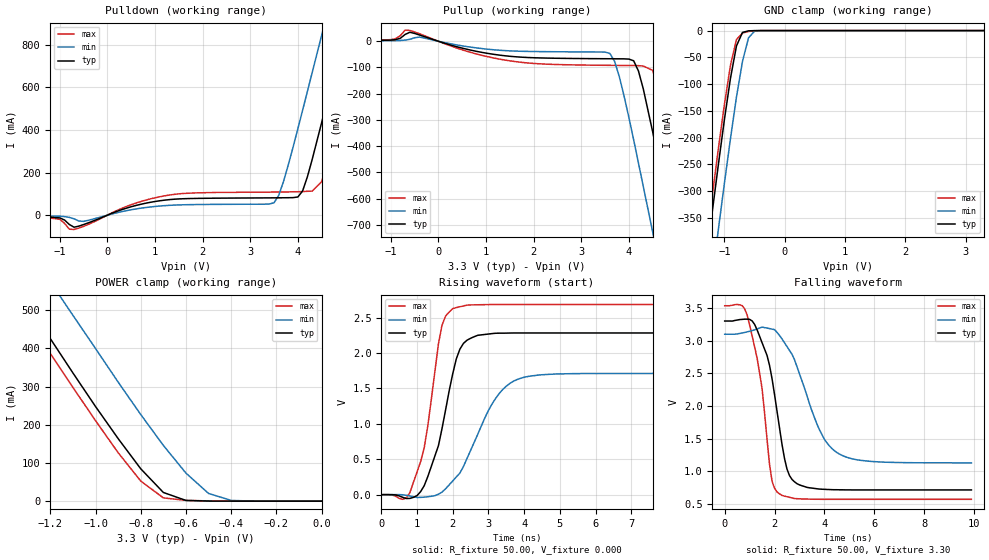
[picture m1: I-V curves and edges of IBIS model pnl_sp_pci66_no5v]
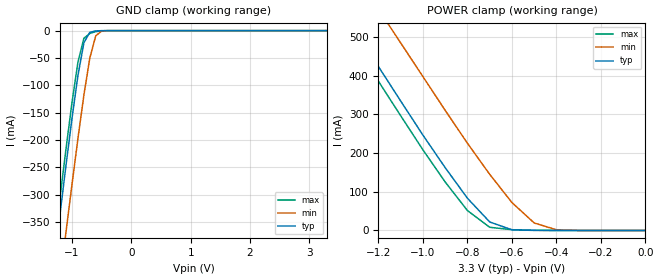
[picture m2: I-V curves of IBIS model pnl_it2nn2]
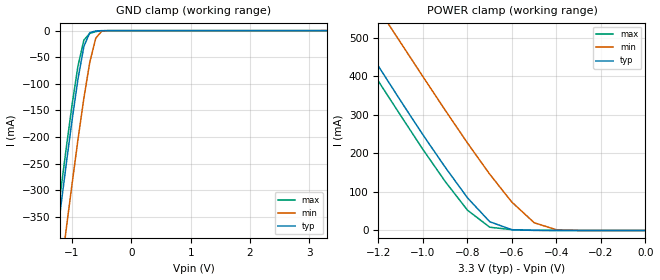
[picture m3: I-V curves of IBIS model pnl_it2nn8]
| IBIS file rc32434.ibs created by s2ibis2 version 1.0
| North Carolina State University Electronics Research Laboratory  1995
| For questions regarding this, please contact senthil:skalidas@idt.com
[IBIS ver]   2.1
[File name]   rc32434.ibs
[File Rev]   1.0
[Date]   July 24, 2003
[Source]   Internetworking Products Division
[Notes]   1. Temperatures: typ=25C, min=0C, max=120C 2. tsmc
0.13lv
   process 3. Ramp rates based on 50 ohm load 4. 1 ohm is
added
   to pad to limit clamp current.
[Disclaimer]   This information is for modeling purposes only, and is
not
   guaranteed.
[Copyright]   Copyright 2002, Integrated Device Technology, Inc.,
All
   Rights are Reserved
|   Component  RC32434
[Component]   rc32434
[Manufacturer]   Integrated Device Technology, Inc.
[Package]
| variable   typ   min   max
R_pkg   0.04   0.02   0.09
L_pkg   4.2nH   3.2nH   7.0nH
C_pkg   0.18pF   0.09pF   0.3pF
[Pin]  signal_name   model_name   R_pin   L_pin
C_pin
A1   rwn   pnl_tf08it0nn2
A2   oen   pnl_tf08it0nn2
B2   rstn   pnl_tf08it0pu2it2nn2
C3   coldrstn   pnl_it2nn8
B1   boen   pnl_tf08it0nn2
C1   extclk   pnl_tf08it0nn2
C2   bdirn   pnl_tf08it0nn2
D2   miicl   pnl_it2pd2
D1   miirxd[00]   pnl_it2pu2
D3   miicrs   pnl_it2pd2
E2   miirxd[02]   pnl_it2pu2
D4   miirxd[01]   pnl_it2pu2
E3   miitxd[00]   pnl_tf08it0nn2
E1   miirxd[03]   pnl_it2pu2
E4   miitxd[01]   pnl_tf08it0nn2
F2   miirxclk   pnl_it2pu2
F1   miitxd[02]   pnl_tf08it0nn2
F3   miitxd[03]   pnl_tf08it0nn2
F4   miitxenp   pnl_tf08it0nn2
G2   miitxer   pnl_tf08it0nn2
G1   miirxdv   pnl_it2pd2
G3   miirxer   pnl_it2pd2
G4   miitxclk   pnl_it2pu2
H2   miimdc   pnl_tf08it0nn2
H1   miimdio   pnl_tf08it0pu2
H3   gpio[00]   pnl_tf08it0pu2
H4   gpio[01]   pnl_tf08it0pu2
J4   ejtag_tms   pnl_it2pu2
J3   gpio[02]   pnl_tf08it0pu2
J1   gpio[03]   pnl_tf08it0pu2
J2   jtag_tck   pnl_it2pu2
K4   sdo   pnl_tf08it0pu2
L4   audisn   pnl_it2nn2
K1   jtag_tdo   pnl_tf08it0nn2
K2   sck   pnl_tf08it0pu2
K3   sdi   pnl_tf08it0pu2
L3   gpio[08]   pnl_tf08it0pu2
L1   sda   pnl_tf08it0pu2it2nn2
L2   scl   pnl_tf08it0pd2it2nn2
M4   gpio[09]   pnl_sp_pci66_no5v
M3   gpio[11]   pnl_sp_pci66_no5v
M1   gpio[12]   pnl_sp_pci66_no5v
M2   pciad[31]   pnl_sp_pci66_no5v
N3   pciad[30]   pnl_sp_pci66_no5v
N1   pciad[29]   pnl_sp_pci66_no5v
N2   pciad[28]   pnl_sp_pci66_no5v
P1   pciad[27]   pnl_sp_pci66_no5v
P2   pciad[26]   pnl_sp_pci66_no5v
R1   pciad[25]   pnl_sp_pci66_no5v
T1   pciad[24]   pnl_sp_pci66_no5v
R2   pcicben[03]   pnl_sp_pci66_no5v
P3   gpio[10]   pnl_sp_pci66_no5v
R3   pciad[23]   pnl_sp_pci66_no5v
T2   gpio[13]   pnl_sp_pci66_no5v
T3   pciad[22]   pnl_sp_pci66_no5v
P4   pciad[20]   pnl_sp_pci66_no5v
R4   pciad[21]   pnl_sp_pci66_no5v
N4   pciad[18]   pnl_sp_pci66_no5v
T4   pciad[19]   pnl_sp_pci66_no5v
R5   pciad[17]   pnl_sp_pci66_no5v
T5   pciad[16]   pnl_sp_pci66_no5v
N5   pcireqn[01]   pnl_sp_pci66_no5v
P5   pcireqn[03]   pnl_sp_pci66_no5v
R6   pcirstn   pnl_sp_pci66_no5v
T6   pciclk   pnl_sp_pci66_no5v
P6   pcireqn[00]   pnl_sp_pci66_no5v
N6   pcireqn[02]   pnl_sp_pci66_no5v
T7   pcigntn[00]   pnl_sp_pci66_no5v
R7   pcicben[02]   pnl_sp_pci66_no5v
P7   pciframen   pnl_sp_pci66_no5v
N7   pciirdyn   pnl_sp_pci66_no5v
R8   pcitrdyn   pnl_sp_pci66_no5v
T8   pcidevseln   pnl_sp_pci66_no5v
P8   pcistopn   pnl_sp_pci66_no5v
N8   pcilockn   pnl_sp_pci66_no5v
N9   pciperrn   pnl_sp_pci66_no5v
P9   pciserrn   pnl_sp_pci66_no5v
T9   pcipar   pnl_sp_pci66_no5v
R9   pcicben[01]   pnl_sp_pci66_no5v
N10   pciad[15]   pnl_sp_pci66_no5v
P10   pciad[14]   pnl_sp_pci66_no5v
T10   pciad[13]   pnl_sp_pci66_no5v
R10   pciad[12]   pnl_sp_pci66_no5v
N11   pciad[11]   pnl_sp_pci66_no5v
P11   pciad[10]   pnl_sp_pci66_no5v
T11   pciad[09]   pnl_sp_pci66_no5v
R11   pciad[08]   pnl_sp_pci66_no5v
N12   pcicben[00]   pnl_sp_pci66_no5v
P12   pciad[07]   pnl_sp_pci66_no5v
T12   pciad[06]   pnl_sp_pci66_no5v
R12   pciad[05]   pnl_sp_pci66_no5v
P13   pciad[04]   pnl_sp_pci66_no5v
R13   pciad[03]   pnl_sp_pci66_no5v
T13   pciad[02]   pnl_sp_pci66_no5v
R14   pciad[00]   pnl_sp_pci66_no5v
T14   pciad[01]   pnl_sp_pci66_no5v
T15   pcigntn[01]   pnl_sp_pci66_no5v
R15   pcigntn[02]   pnl_sp_pci66_no5v
T16   pcigntn[03]   pnl_sp_pci66_no5v
P14   ddraddr[00]   pnl_sstl_2classi
R16   ddraddr[01]   pnl_sstl_2classi
P15   ddraddr[02]   pnl_sstl_2classi
N15   ddraddr[03]   pnl_sstl_2classi
P16   ddrcsn   pnl_sstl_2classi
N14   ddraddr[04]   pnl_sstl_2classi
N16   ddrba[00]   pnl_sstl_2classi
N13   ddraddr[05]   pnl_sstl_2classi
M14   ddrba[01]   pnl_sstl_2classi
M15   ddraddr[06]   pnl_sstl_2classi
M16   ddraddr[07]   pnl_sstl_2classi
M13   ddrrasn   pnl_sstl_2classi
L15   ddrcasn   pnl_sstl_2classi
L14   ddrwen   pnl_sstl_2classi
L16   ddraddr[08]   pnl_sstl_2classi
L13   ddraddr[09]   pnl_sstl_2classi
K15   ddraddr[10]   pnl_sstl_2classi
K14   ddraddr[11]   pnl_sstl_2classi
K16   ddraddr[12]   pnl_sstl_2classi
K13   ddrcke   pnl_sstl_2classi
J15   ddrckp   pnl_sstl_2classi
J16   ddrdqs[00]   pnl_sstl_2classi
J13   ddrckn   pnl_sstl_2classi
H13   ddrdata[15]   pnl_sstl_2classi
H14   ddrdata[14]   pnl_sstl_2classi
H16   ddrdata[13]   pnl_sstl_2classi
G13   ddrdm[01]   pnl_sstl_2classi
G14   ddrdqs[01]   pnl_sstl_2classi
G16   ddrdata[11]   pnl_sstl_2classi
G15   ddrdata[10]   pnl_sstl_2classi
F13   ddrdata[09]   pnl_sstl_2classi
F14   ddrdata[08]   pnl_sstl_2classi
F16   ddrdata[07]   pnl_sstl_2classi
F15   ddrdm[00]   pnl_sstl_2classi
E13   ddrdata[06]   pnl_sstl_2classi
E14   ddrdata[05]   pnl_sstl_2classi
E16   ddrdata[04]   pnl_sstl_2classi
E15   ddraddr[13]   pnl_sstl_2classi
D15   ddrdata[03]   pnl_sstl_2classi
D14   ddrdata[02]   pnl_sstl_2classi
D16   ddrdata[01]   pnl_sstl_2classi
C16   ddrdata[00]   pnl_sstl_2classi
C15   maddr[00]   pnl_tf08it0nn2
B16   maddr[01]   pnl_tf08it0nn2
A16   maddr[02]   pnl_tf08it0nn2
B15   maddr[03]   pnl_tf08it0nn2
A15   maddr[05]   pnl_tf08it0nn2
C14   maddr[04]   pnl_tf08it0nn2
B14   maddr[06]   pnl_tf08it0nn2
B13   maddr[08]   pnl_tf08it0nn2
A14   maddr[07]   pnl_tf08it0nn2
A13   maddr[09]   pnl_tf08it0nn2
C13   clk   pnl_it2nn8
D13   waitackn   pnl_it2pu2
D12   jtag_trstn   pnl_it2pu2
A12   jtag_tdi   pnl_it2pu2
C11   jtag_tms   pnl_it2pu2
D11   extbcv   pnl_it2pu2
B10   maddr[12]   pnl_tf08it0nn2
A10   maddr[13]   pnl_tf08it0nn2
C10   maddr[14]   pnl_tf08it0nn2
D10   maddr[15]   pnl_tf08it0nn2
A9   maddr[16]   pnl_tf08it0nn2
B9   maddr[17]   pnl_tf08it0nn2
C9   maddr[18]   pnl_tf08it0nn2
D9   maddr[19]   pnl_tf08it0nn2
D8   maddr[20]   pnl_tf08it0nn2
C8   maddr[21]   pnl_tf08it0nn2
A8   gpio[04]   pnl_tf08it0pu2
B8   gpio[05]   pnl_tf08it0pu2
C7   gpio[06]   pnl_tf08it0pu2
D7   mdata[00]   pnl_tf08it0nn2
B7   mdata[04]   pnl_tf08it0nn2
A7   gpio[07]   pnl_tf08it0pu2
C6   mdata[05]   pnl_tf08it0nn2
D6   mdata[02]   pnl_tf08it0nn2
A6   mdata[06]   pnl_tf08it0nn2
B6   mdata[01]   pnl_tf08it0nn2
D5   mdata[07]   pnl_tf08it0nn2
A5   maddr[10]   pnl_tf08it0nn2
C5   mdata[03]   pnl_tf08it0nn2
B5   maddr[11]   pnl_tf08it0nn2
C4   wen   pnl_tf08it0nn2
B4   csn[01]   pnl_tf08it0nn2
A4   csn[00]   pnl_tf08it0nn2
A3   csn[02]   pnl_tf08it0nn2
B3   csn[03]   pnl_tf08it0nn2
|in   IN   DUMMY_MODEL
|oe   OE   DUMMY_MODEL
|   Model pnl_sp_pci66_no5v
| Models and submodels in the file (10): pnl_sp_pci66_no5v (I/O), pnl_it2nn2 (Input), pnl_it2nn8 (Input), pnl_it2pd2 (Input), pnl_it2pu2 (Input), pnl_tf08it0nn2 (I/O), pnl_tf08it0pd2it2nn2 (I/O), pnl_tf08it0pu2 (I/O), pnl_tf08it0pu2it2nn2 (I/O), pnl_sstl_2classi (I/O)
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[Model]   pnl_sp_pci66_no5v
Model_type   I/O
Polarity   Non-Inverting
Enable   Active-High
Vinl =  0.800V
Vinh =  2.000V
Vmeas =  1.500V
C_comp   0.40pF   0.30pF   0.50pF
[Temperature Range]   25.00   0.12k   0.000
[Voltage Range]   3.30V   3.00V   3.60V
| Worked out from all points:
|   slope of the pulldown table from 0 to 0.495 V, typ, clamps not added: 12.6 ohm
|   slope of the pullup table from 0 to 0.495 V, typ, clamps not added: 19.1 ohm
|   GND clamp passes 1 mA (typ) near -0.62 V on its own axis
|   POWER clamp passes 1 mA (typ) near -0.55 V on its own axis
|   rising waveform, R_fixture 50.00, V_fixture 0.000: 20-80 % time 618ps typ, 976ps min, 470ps max; typ from 0 V to 2.28 V
|   falling waveform, R_fixture 50.00, V_fixture 3.30: 20-80 % time 695ps typ, 1.15ns min, 606ps max; typ from 3.3 V to 0.714 V
[Pulldown]
| voltage   I(typ)   I(min)   I(max)
-3.3V     -4mA       -4mA       -5mA
-700mV    -56.54mA   -17.25mA   -67.28mA
1.1V      67.59mA    42.9mA     86.43mA
3.4V      81.21mA    52.14mA    108mA
3.6V      81.5mA     93.93mA    109mA
4V        85.29mA    406mA      110mA
4.2V      180mA      581mA      112mA
4.5V      435mA      845mA      157mA
4.9V      793mA      1.196A     489mA
5.1V      973mA      1.373A     669mA
5.3V      1.152A     1.549A     850mA
6.6V      2.322A     2.695A     2.025A
[Pullup]
| voltage   I(typ)   I(min)   I(max)
-3.3V     3mA        2mA        3mA
-1V       4.3mA      2.1mA      6.2mA
-600mV    34.47mA    7.44mA     41.38mA
1.3V      -53.2mA    -34.37mA   -68.6mA
3.6V      -66.65mA   -46.33mA   -91.8mA
3.8V      -66.85mA   -136mA     -92.09mA
4.1V      -74.41mA   -376mA     -92.5mA
4.3V      -180mA     -552mA     -94.45mA
4.5V      -346mA     -728mA     -111mA
4.9V      -704mA     -1.082A    -406mA
5.3V      -1.064A    -1.436A    -767mA
6.6V      -2.239A    -2.587A    -1.948A
[GND_clamp]
| voltage   I(typ)   I(min)   I(max)
-3.3V     -2.233A    -2.317A    -2.212A
-1.3V     -427mA     -547mA     -396mA
-1.2V     -337mA     -459mA     -307mA
-1.1V     -250mA     -371mA     -220mA
-1V       -166mA     -285mA     -138mA
-900mV    -89.23mA   -202mA     -64.85mA
-800mV    -28.56mA   -124mA     -16.52mA
-700mV    -3.449mA   -57.38mA   -4.708mA
-600mV    -516uA     -13.49mA   -1.622mA
-500mV    -73.1uA    -1.086mA   -307uA
3.3V      236pA      104uA      0A
[POWER_clamp]
| voltage   I(typ)   I(min)   I(max)
-3.3V     2.314A     2.425A     2.286A
-1.4V     605mA      750mA      568mA
-1.3V     515mA      663mA      477mA
-1.2V     426mA      575mA      387mA
-1.1V     336mA      487mA      298mA
-900mV    164mA      312mA      127mA
-800mV    84.75mA    227mA      52.71mA
-700mV    22.7mA     146mA      8.493mA
-600mV    1.787mA    73.39mA    1.962mA
-500mV    198uA      20.05mA    609uA
-400mV    23.19uA    1.835mA    90.11uA
0V        255pA      438pA      -934pA
[Ramp]
| variable   typ   min   max
dV/dt_r   1.37/0.62n   1.03/0.98n   1.61/0.47n
dV/dt_f   1.55/0.69n   1.21/1.18n   1.78/0.59n
R_load = 50.00
[Rising Waveform]
R_fixture = 50.00
V_fixture = 0.000
| time   V(typ)   V(min)   V(max)
0s        111uV      95.81uV    134uV
800ps     -52.97mV   -17.77mV   29.66mV
1.2ns     125mV      -35.3mV    659mV
1.6ns     692mV      6.094mV    2.13V
1.8ns     1.197V     82.88mV    2.522V
2ns       1.707V     194mV      2.627V
2.4ns     2.181V     511mV      2.676V
3.1ns     2.274V     1.28V      2.684V
3.8ns     2.283V     1.625V     2.685V
9.9ns     2.283V     1.711V     2.685V
[Falling Waveform]
R_fixture = 50.00
V_fixture = 3.30
| time   V(typ)   V(min)   V(max)
0s        3.3V       3.098V     3.534V
900ps     3.329V     3.134V     3.395V
1.4ns     3.067V     3.193V     2.505V
1.7ns     2.772V     3.192V     1.485V
1.9ns     2.416V     3.176V     848mV
2.1ns     1.918V     3.126V     683mV
2.7ns     875mV      2.792V     591mV
3.8ns     727mV      1.637V     571mV
4.5ns     717mV      1.287V     570mV
9.9ns     714mV      1.128V     570mV
[Model]   pnl_it2nn2
Model_type   Input
Polarity   Non-Inverting
Enable   Active-High
Vinl =  0.800V
Vinh =  2.000V
C_comp   0.40pF   0.30pF   0.50pF
[Temperature Range]   25.00   0.12k   0.000
[Voltage Range]   3.30V   3.00V   3.60V
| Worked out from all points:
|   GND clamp passes 1 mA (typ) near -0.62 V on its own axis
|   POWER clamp passes 1 mA (typ) near -0.55 V on its own axis
[GND_clamp]
| voltage   I(typ)   I(min)   I(max)
-3.3V     -2.227A    -2.314A    -2.206A
-1.3V     -423mA     -544mA     -392mA
-1.2V     -333mA     -455mA     -303mA
-1.1V     -245mA     -367mA     -215mA
-1V       -160mA     -281mA     -131mA
-900mV    -81.93mA   -197mA     -57.56mA
-800mV    -22.3mA    -118mA     -14.01mA
-700mV    -2.961mA   -50.16mA   -5.175mA
-600mV    -550uA     -9.434mA   -1.81mA
-500mV    -66.25uA   -683uA     -324uA
3.3V      208pA      98.6uA     -311pA
[POWER_clamp]
| voltage   I(typ)   I(min)   I(max)
-3.3V     2.297A     2.407A     2.27A
-1.4V     601mA      745mA      564mA
-1.3V     512mA      658mA      474mA
-1.2V     423mA      571mA      385mA
-1.1V     334mA      484mA      296mA
-900mV    162mA      310mA      125mA
-800mV    83.1mA     225mA      51.35mA
-700mV    21.93mA    145mA      8.218mA
-600mV    1.732mA    71.99mA    1.948mA
-500mV    190uA      19.39mA    600uA
-400mV    17.43uA    1.765mA    83.01uA
0V        208pA      441pA      -973pA
[Model]   pnl_it2nn8
Model_type   Input
Polarity   Non-Inverting
Enable   Active-High
Vinl =  0.800V
Vinh =  2.000V
C_comp   0.40pF   0.30pF   0.50pF
[Temperature Range]   25.00   0.12k   0.000
[Voltage Range]   3.30V   3.00V   3.60V
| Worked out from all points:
|   GND clamp passes 1 mA (typ) near -0.61 V on its own axis
|   POWER clamp passes 1 mA (typ) near -0.55 V on its own axis
[GND_clamp]
| voltage   I(typ)   I(min)   I(max)
-3.3V     -2.251A    -2.341A    -2.23A
-1.3V     -430mA     -553mA     -400mA
-1.2V     -341mA     -464mA     -310mA
-1.1V     -253mA     -375mA     -223mA
-1V       -169mA     -289mA     -140mA
-900mV    -91.2mA    -205mA     -66.62mA
-800mV    -29.65mA   -127mA     -17.63mA
-700mV    -3.751mA   -59.22mA   -5.273mA
-600mV    -566uA     -14.16mA   -1.811mA
-500mV    -66.52uA   -1.151mA   -324uA
3.3V      428pA      101uA      -47.08pA
[POWER_clamp]
| voltage   I(typ)   I(min)   I(max)
-3.3V     2.315A     2.426A     2.287A
-1.4V     605mA      750mA      568mA
-1.3V     515mA      662mA      477mA
-1.2V     426mA      575mA      387mA
-1.1V     336mA      487mA      298mA
-900mV    164mA      312mA      127mA
-800mV    84.72mA    227mA      52.68mA
-700mV    22.75mA    146mA      8.48mA
-600mV    1.78mA     73.35mA    1.952mA
-500mV    191uA      20.03mA    600uA
-400mV    17.44uA    1.832mA    83.02uA
0V        428pA      1.015nA    -667pA
